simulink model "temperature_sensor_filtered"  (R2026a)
settings: Solver=FixedStepAuto  StopTime=inf  EnableMultiTasking=on
undefined symbols (not defined in the file): dspblkCoreblockFVToolHelper, gcbh
libraries: arduinolib x1

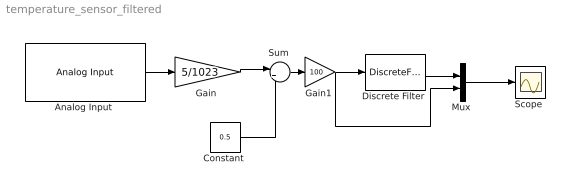
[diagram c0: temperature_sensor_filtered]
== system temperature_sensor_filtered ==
  "Analog Input " : arduinolib/Analog Input  pinNumber=4  ReadResultsOnly=off  ConversionTriggerSource=Software  ExternalTriggerType=uint32( 0 )  OutputDataType=uint16  EnableConversionCompleteNotify=off  EnableOuputStatus=off  SampleTime=0.01  blockPlatform=arduino
  "Constant " : Constant  Value=0.5
  "Discrete Filter " : DiscreteFilter  LoadFcn=dspblkCoreblockFVToolHelper(gcbh,'load');  Numerator=[0.00995]  Denominator=[1 -0.99]
  "Gain " : Gain  Gain=5/1023
  "Gain1 " : Gain  Gain=100
  "Mux " : Mux  Inputs=2
  "Scope " : Scope
  "Sum " : Sum  Inputs=|+-
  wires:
  "Analog Input "/1 -> "Gain "/1
  "Gain "/1 -> "Sum "/1
  "Constant "/1 -> "Sum "/2
  "Sum "/1 -> "Gain1 "/1
  "Mux "/1 -> "Scope "/1
  "Gain1 "/1 -> "Mux "/2, "Discrete Filter "/1
  "Discrete Filter "/1 -> "Mux "/1
